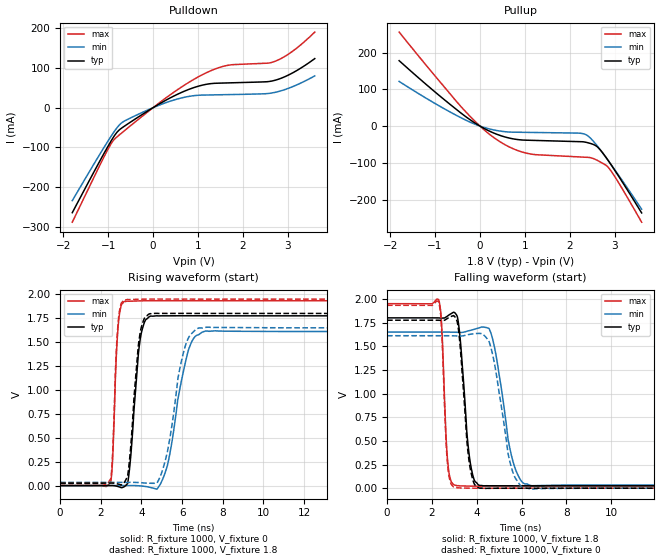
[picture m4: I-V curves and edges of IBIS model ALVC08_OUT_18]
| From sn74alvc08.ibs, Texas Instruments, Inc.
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[Model]   ALVC08_OUT_18
Model_type  Output
Vref =   0
Rref =   1000
Cref =   30p
Vmeas =   0.9
| variable   typ   min   max
C_comp   8.44pF   5.76pF   11.61pF
| C_pullup   8.55pF   6.36pF   9.47pF
| C_pulldown   8.32pF   5.76pF   11.61pF
[Temperature Range]   40   100   -40
| Ambient temperature   25   85   -40
[Voltage range]   1.8   1.65   1.95
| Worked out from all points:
|   slope of the pulldown table from 0 to 0.27 V, typ, clamps not added: 15.1 ohm
|   slope of the pullup table from 0 to 0.27 V, typ, clamps not added: 15.9 ohm
|   rising waveform, R_fixture 1000, V_fixture 0: 20-80 % time 379ps typ, 776ps min, 210ps max; typ from 0 V to 1.77 V
|   falling waveform, R_fixture 1000, V_fixture 1.8: 20-80 % time 339ps typ, 621ps min, 198ps max; typ from 1.8 V to 0.026 V
|   rising waveform, R_fixture 1000, V_fixture 1.8: 20-80 % time 377ps typ, 714ps min, 208ps max; typ from 0.026 V to 1.8 V
|   falling waveform, R_fixture 1000, V_fixture 0: 20-80 % time 335ps typ, 624ps min, 196ps max; typ from 1.77 V to 0 V
[Pulldown]
| ALVC08_OUT_18
|   Voltage   I(typ)   I(min)   I(max)
-1.8V     -264.5mA   -234.1mA   -288.3mA
-1.155V   -127.9mA   -111.4mA   -137.9mA
-915mV    -80.08mA   -68.36mA   -87.27mA
-800mV    -61.37mA   -50.08mA   -73.15mA
-690mV    -50.59mA   -37.38mA   -62.82mA
-210mV    -14.85mA   -10.42mA   -18.81mA
550mV     34.08mA    22.06mA    45.73mA
1.16V     58.24mA    31.77mA    86.5mA
1.675V    62.35mA    32.87mA    106.8mA
2.71V     68.82mA    38.41mA    116.5mA
3.115V    88.05mA    53.24mA    142.8mA
3.6V      123.5mA    79.91mA    190.3mA
[Pullup]
| ALVC08_OUT_18
|   Voltage   I(typ)   I(min)   I(max)
-1.8V     177.9mA    121.4mA    255.7mA
-380mV    31.41mA    20.06mA    47.26mA
40mV      -2.839mA   -1.667mA   -4.509mA
390mV     -22.94mA   -12.43mA   -38.14mA
740mV     -34.79mA   -16.58mA   -61.65mA
1.095V    -38.57mA   -17.2mA    -75.19mA
2.195V    -42.3mA    -19.18mA   -83.81mA
2.365V    -44.23mA   -23.75mA   -84.88mA
2.61V     -56.21mA   -53.66mA   -93.1mA
2.865V    -95.44mA   -95.17mA   -113.5mA
3.105V    -139.7mA   -136.8mA   -157.6mA
3.6V      -236.1mA   -226.1mA   -261.5mA
[Ramp]
| ALVC08_OUT_18
| variable   typ   min   max
dV/dt_r   1.08/4.30E-10   0.99/8.39E-10   1.17/2.18E-10
dV/dt_f   1.10/3.91E-10   1.00/7.22E-10   1.19/2.17E-10
R_load = 1000
[Rising Waveform]
| ALVC08_OUT_18
R_fixture =   1000
C_fixture =   0
L_fixture =   0
V_fixture =   0
V_fixture_min = 0
V_fixture_max = 0
|   Time   V(typ)   V(min)   V(max)
0s        30.49pV    5.701nV    21.71pV
2.5ns     952.9uV    454.8uV    44.05mV
2.845ns   -9.601mV   557.5uV    1.645V
3.165ns   -9.371mV   508.4uV    1.926V
3.41ns    169.9mV    483.5uV    1.928V
3.94ns    1.533V     -3.269mV   1.932V
4.46ns    1.773V     -20.22mV   1.933V
6.34ns    1.776V     1.435V     1.933V
7.135ns   1.776V     1.615V     1.933V
50ns      1.775V     1.611V     1.933V
[Falling Waveform]
| ALVC08_OUT_18
R_fixture =   1000
C_fixture =   0
L_fixture =   0
V_fixture =   1.8
V_fixture_min = 1.65
V_fixture_max = 1.95
|   Time   V(typ)   V(min)   V(max)
0s        1.8V       1.65V      1.95V
2.305ns   1.799V     1.65V      1.992V
2.72ns    1.823V     1.65V      250.2mV
3.11ns    1.827V     1.648V     27.14mV
3.68ns    325.1mV    1.665V     22.37mV
4.135ns   28.52mV    1.697V     21.38mV
4.72ns    26.05mV    1.568V     21.27mV
5.69ns    25.08mV    226.6mV    21.6mV
6.46ns    25.29mV    26.28mV    21.73mV
50ns      25.59mV    33.88mV    21.73mV
[Rising Waveform]
| ALVC08_OUT_18
R_fixture =   1000
C_fixture =   0
L_fixture =   0
V_fixture =   1.8
V_fixture_min = 1.65
V_fixture_max = 1.95
|   Time   V(typ)   V(min)   V(max)
0s        25.59mV    33.88mV    21.73mV
2.5ns     26.34mV    34.32mV    77.46mV
2.82ns    17.7mV     34.3mV     1.616V
3.155ns   33.89mV    34.11mV    1.942V
3.395ns   230.9mV    33.98mV    1.945V
3.91ns    1.565V     31.39mV    1.949V
4.425ns   1.798V     24.63mV    1.95V
6.155ns   1.801V     1.46V      1.95V
6.855ns   1.8V       1.649V     1.95V
50ns      1.8V       1.65V      1.95V
[Falling Waveform]
| ALVC08_OUT_18
R_fixture =   1000
C_fixture =   0
L_fixture =   0
V_fixture =   0
V_fixture_min = 0
V_fixture_max = 0
|   Time   V(typ)   V(min)   V(max)
0s        1.775V     1.611V     1.933V
2.305ns   1.775V     1.611V     1.968V
2.43ns    1.774V     1.611V     1.707V
2.7ns     1.794V     1.611V     254.8mV
3.105ns   1.777V     1.609V     4.865mV
3.66ns    287.3mV    1.625V     679.5uV
4.125ns   696.6uV    1.636V     -335.5uV
4.61ns    -1.052mV   1.507V     -515uV
6.145ns   -392.7uV   -1.067mV   -35.21uV
50ns      31.67pV    157.5pV    21.92pV
